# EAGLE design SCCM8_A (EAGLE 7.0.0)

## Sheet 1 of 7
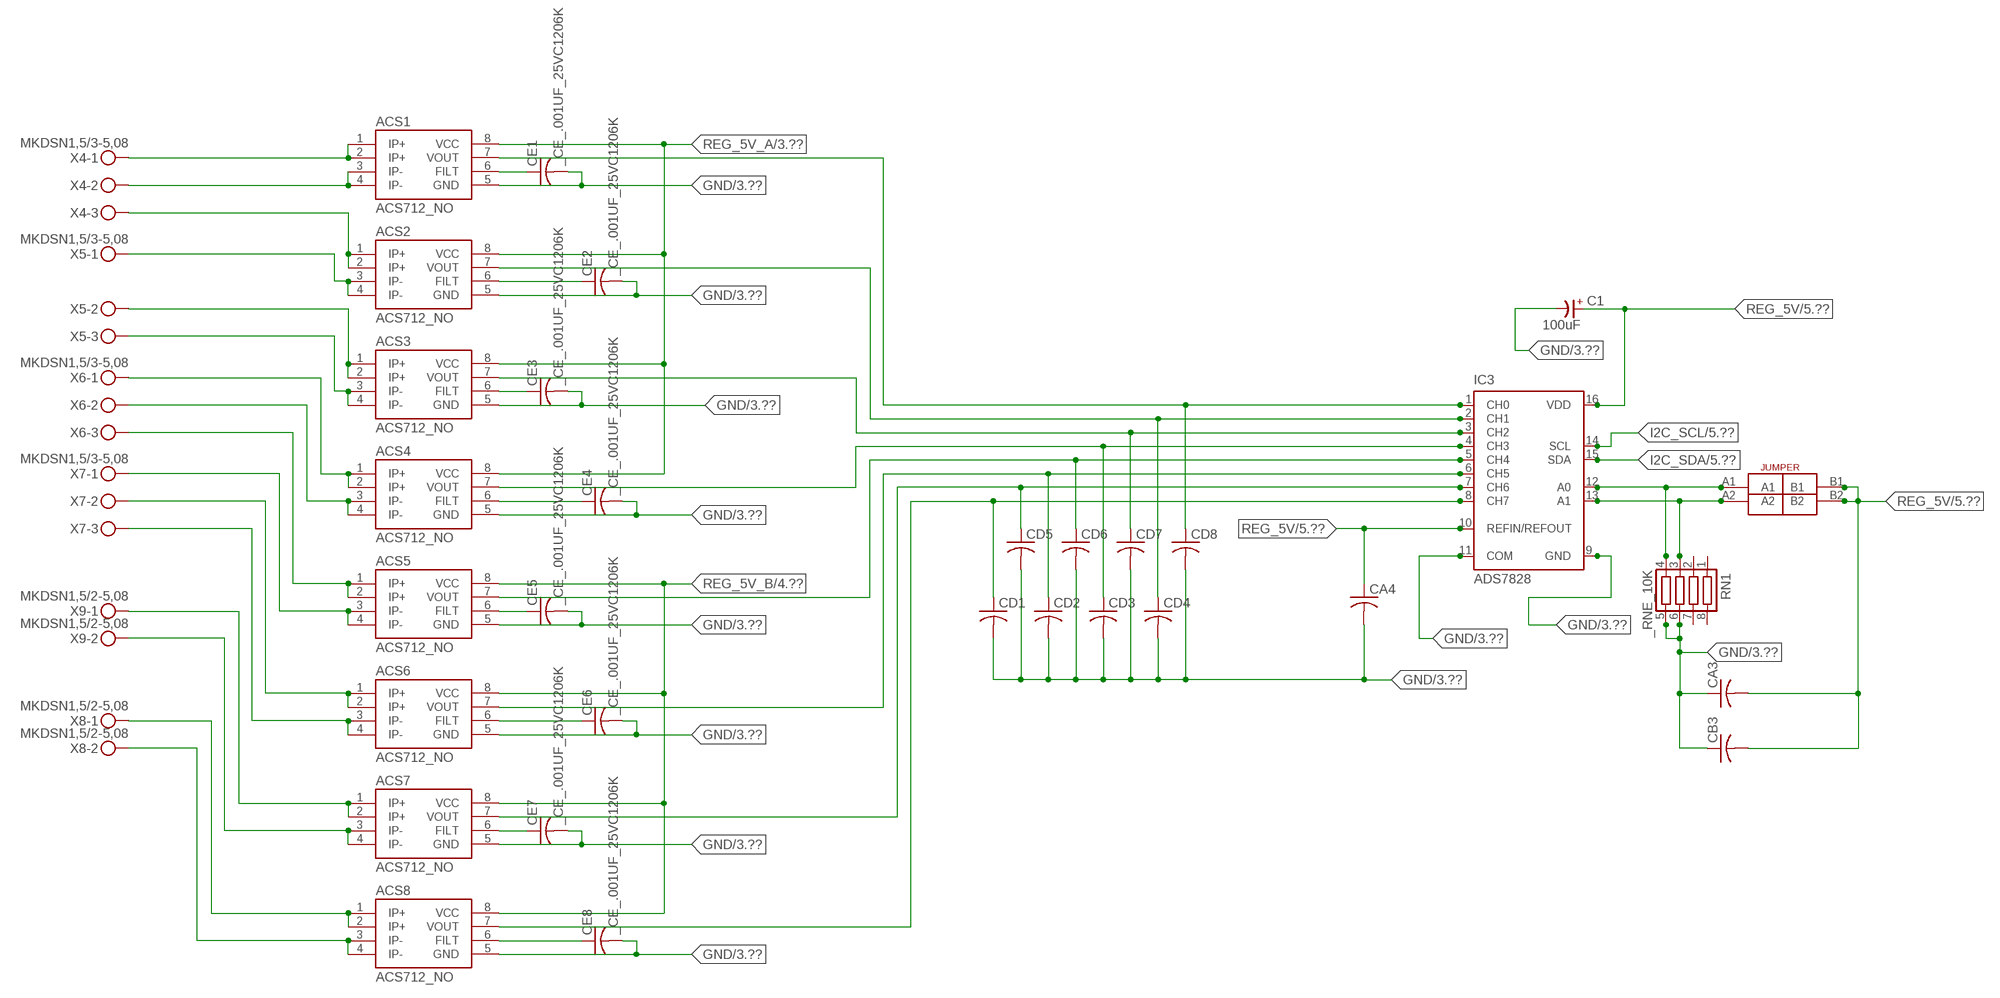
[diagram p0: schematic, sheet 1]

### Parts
ACS1  ACS712_NO  [_MA_DUAL_N-FET]
ACS2  ACS712_NO  [_MA_DUAL_N-FET]
ACS3  ACS712_NO  [_MA_DUAL_N-FET]
ACS4  ACS712_NO  [_MA_DUAL_N-FET]
ACS5  ACS712_NO  [_MA_DUAL_N-FET]
ACS6  ACS712_NO  [_MA_DUAL_N-FET]
ACS7  ACS712_NO  [_MA_DUAL_N-FET]
ACS8  ACS712_NO  [_MA_DUAL_N-FET]
C1  100uF  CP-E-025X060  [E-025X060]
CA3  CC1206KRX7R9BB104C1206K  [CC1206KRX7R9BB104]
CA4  CC1206KRX7R9BB104C1206K  [CC1206KRX7R9BB104]
CB3  TMK316F106ZL-TC1206K  [TMK316F106ZL-T]
CD1  _CD_10NF_50VC1206K  [_CD_10NF_50V]
CD2  _CD_10NF_50VC1206K  [_CD_10NF_50V]
CD3  _CD_10NF_50VC1206K  [_CD_10NF_50V]
CD4  _CD_10NF_50VC1206K  [_CD_10NF_50V]
CD5  _CD_10NF_50VC1206K  [_CD_10NF_50V]
CD6  _CD_10NF_50VC1206K  [_CD_10NF_50V]
CD7  _CD_10NF_50VC1206K  [_CD_10NF_50V]
CD8  _CD_10NF_50VC1206K  [_CD_10NF_50V]
CE1  _CE_.001UF_25VC1206K  [CE]
CE2  _CE_.001UF_25VC1206K  [CE]
CE3  _CE_.001UF_25VC1206K  [CE]
CE4  _CE_.001UF_25VC1206K  [CE]
CE5  _CE_.001UF_25VC1206K  [CE]
CE6  _CE_.001UF_25VC1206K  [CE]
CE7  _CE_.001UF_25VC1206K  [CE]
CE8  _CE_.001UF_25VC1206K  [CE]
IC3  ADS7828  [TSSOP16-PW]
RN1  _RNE_10K  [RNE]
U$4  JUMPER_2X2  [JUMPER_2X2]
X4  MKDSN1,5/3-5,08  [MKDSN1,5/3-5,08]
X5  MKDSN1,5/3-5,08  [MKDSN1,5/3-5,08]
X6  MKDSN1,5/3-5,08  [MKDSN1,5/3-5,08]
X7  MKDSN1,5/3-5,08  [MKDSN1,5/3-5,08]
X8  MKDSN1,5/2-5,08  [MKDSN1,5/2-5,08]
X9  MKDSN1,5/2-5,08  [MKDSN1,5/2-5,08]

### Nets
GND: ACS1.5(GND) ACS2.5(GND) ACS3.5(GND) ACS4.5(GND) ACS5.5(GND) ACS6.5(GND) ACS7.5(GND) ACS8.5(GND) C1.- CA3.1 CA4.2 CB3.1 CD1.2 CD2.2 CD3.2 CD4.2 CD5.2 CD6.2 CD7.2 CD8.2 CE1.2 CE2.2 CE3.2 CE4.2 CE5.2 CE6.2 CE7.2 CE8.2 IC3.9(GND) IC3.11(COM) RN1.5 RN1.6 ; also sheet 3,4,5,7
I2C_SCL: IC3.14(SCL) ; also sheet 5
I2C_SDA: IC3.15(SDA) ; also sheet 5
N$6: ACS5.7(VOUT) CD6.1 IC3.5(CH4)
N$7: ACS1.1(IP+) ACS1.2(IP+) X4.1
N$8: ACS1.3(IP-) ACS1.4(IP-) X4.2
N$9: ACS1.7(VOUT) CD8.1 IC3.1(CH0)
N$10: ACS2.7(VOUT) CD4.1 IC3.2(CH1)
N$11: ACS3.7(VOUT) CD7.1 IC3.3(CH2)
N$12: ACS4.7(VOUT) CD3.1 IC3.4(CH3)
N$13: ACS2.1(IP+) ACS2.2(IP+) X4.3
N$14: ACS6.7(VOUT) CD2.1 IC3.6(CH5)
N$15: ACS7.7(VOUT) CD5.1 IC3.7(CH6)
N$16: ACS2.3(IP-) ACS2.4(IP-) X5.1
N$17: IC3.12(A0) RN1.4 U$4.A1
N$18: IC3.13(A1) RN1.3 U$4.A2
N$19: ACS3.1(IP+) ACS3.2(IP+) X5.2
N$20: ACS3.3(IP-) ACS3.4(IP-) X5.3
N$21: ACS4.1(IP+) ACS4.2(IP+) X6.1
N$22: ACS4.3(IP-) ACS4.4(IP-) X6.2
N$23: ACS5.1(IP+) ACS5.2(IP+) X6.3
N$24: ACS5.3(IP-) ACS5.4(IP-) X7.1
N$25: ACS6.1(IP+) ACS6.2(IP+) X7.2
N$26: ACS6.3(IP-) ACS6.4(IP-) X7.3
N$27: ACS7.1(IP+) ACS7.2(IP+) X9.1
N$28: ACS7.3(IP-) ACS7.4(IP-) X9.2
N$29: ACS8.1(IP+) ACS8.2(IP+) X8.1
N$30: ACS8.3(IP-) ACS8.4(IP-) X8.2
N$33: ACS1.6(FILT) CE1.1
N$34: ACS2.6(FILT) CE2.1
N$35: ACS3.6(FILT) CE3.1
N$36: ACS4.6(FILT) CE4.1
N$37: ACS8.7(VOUT) CD1.1 IC3.8(CH7)
N$38: ACS5.6(FILT) CE5.1
N$39: ACS6.6(FILT) CE6.1
N$40: ACS7.6(FILT) CE7.1
N$41: ACS8.6(FILT) CE8.1
REG_5V: C1.+ CA3.2 CA4.1 CB3.2 IC3.10(REFIN/REFOUT) IC3.16(VDD) U$4.B1 U$4.B2 ; also sheet 5,7
REG_5V_A: ACS1.8(VCC) ACS2.8(VCC) ACS3.8(VCC) ACS4.8(VCC) ; also sheet 3
REG_5V_B: ACS5.8(VCC) ACS6.8(VCC) ACS7.8(VCC) ACS8.8(VCC) ; also sheet 4
Unconnected: RN1.1 RN1.2 RN1.7 RN1.8

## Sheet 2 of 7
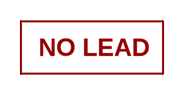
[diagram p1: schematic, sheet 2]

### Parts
U$16  NOPB_LOGO_SYM  [NOPB_LOGO_SYM]

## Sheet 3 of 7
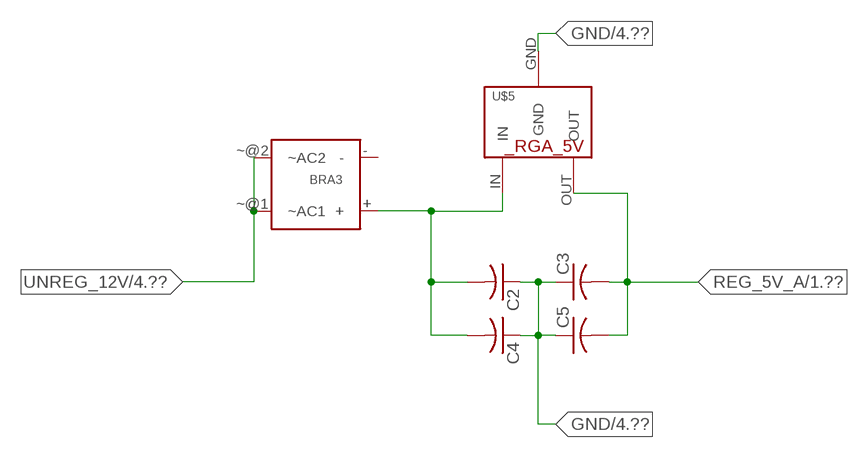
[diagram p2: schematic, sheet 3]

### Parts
BRA3  MB2S_  [MB2S]
C2  _CA_.10UF_50VC1206K  [_CA_.1UF_50V]
C3  _CA_.10UF_50VC1206K  [_CA_.1UF_50V]
C4  _CB_10UF_25VC1206K  [_CB_10UF_25V]
C5  _CB_10UF_25VC1206K  [_CB_10UF_25V]
U$5  _RGA_5V  [_RGA_5V]

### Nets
GND: C2.1 C3.1 C4.1 C5.1 U$5.GND ; also sheet 1,4,5,7
N$31: BRA3.+ C2.2 C4.2 U$5.IN
REG_5V_A: C3.2 C5.2 U$5.OUT ; also sheet 1
UNREG_12V: BRA3.~@1(~AC1) BRA3.~@2(~AC2) ; also sheet 4,5
Unconnected: BRA3.-

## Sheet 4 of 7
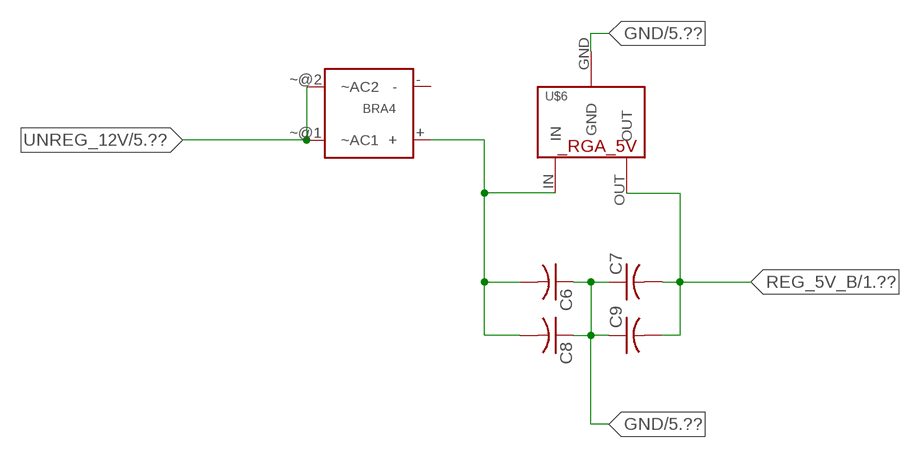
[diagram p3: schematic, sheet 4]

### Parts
BRA4  MB2S_  [MB2S]
C6  _CA_.10UF_50VC1206K  [_CA_.1UF_50V]
C7  _CA_.10UF_50VC1206K  [_CA_.1UF_50V]
C8  _CB_10UF_25VC1206K  [_CB_10UF_25V]
C9  _CB_10UF_25VC1206K  [_CB_10UF_25V]
U$6  _RGA_5V  [_RGA_5V]

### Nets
GND: C6.1 C7.1 C8.1 C9.1 U$6.GND ; also sheet 1,3,5,7
N$32: BRA4.+ C6.2 C8.2 U$6.IN
REG_5V_B: C7.2 C9.2 U$6.OUT ; also sheet 1
UNREG_12V: BRA4.~@1(~AC1) BRA4.~@2(~AC2) ; also sheet 3,5
Unconnected: BRA4.-

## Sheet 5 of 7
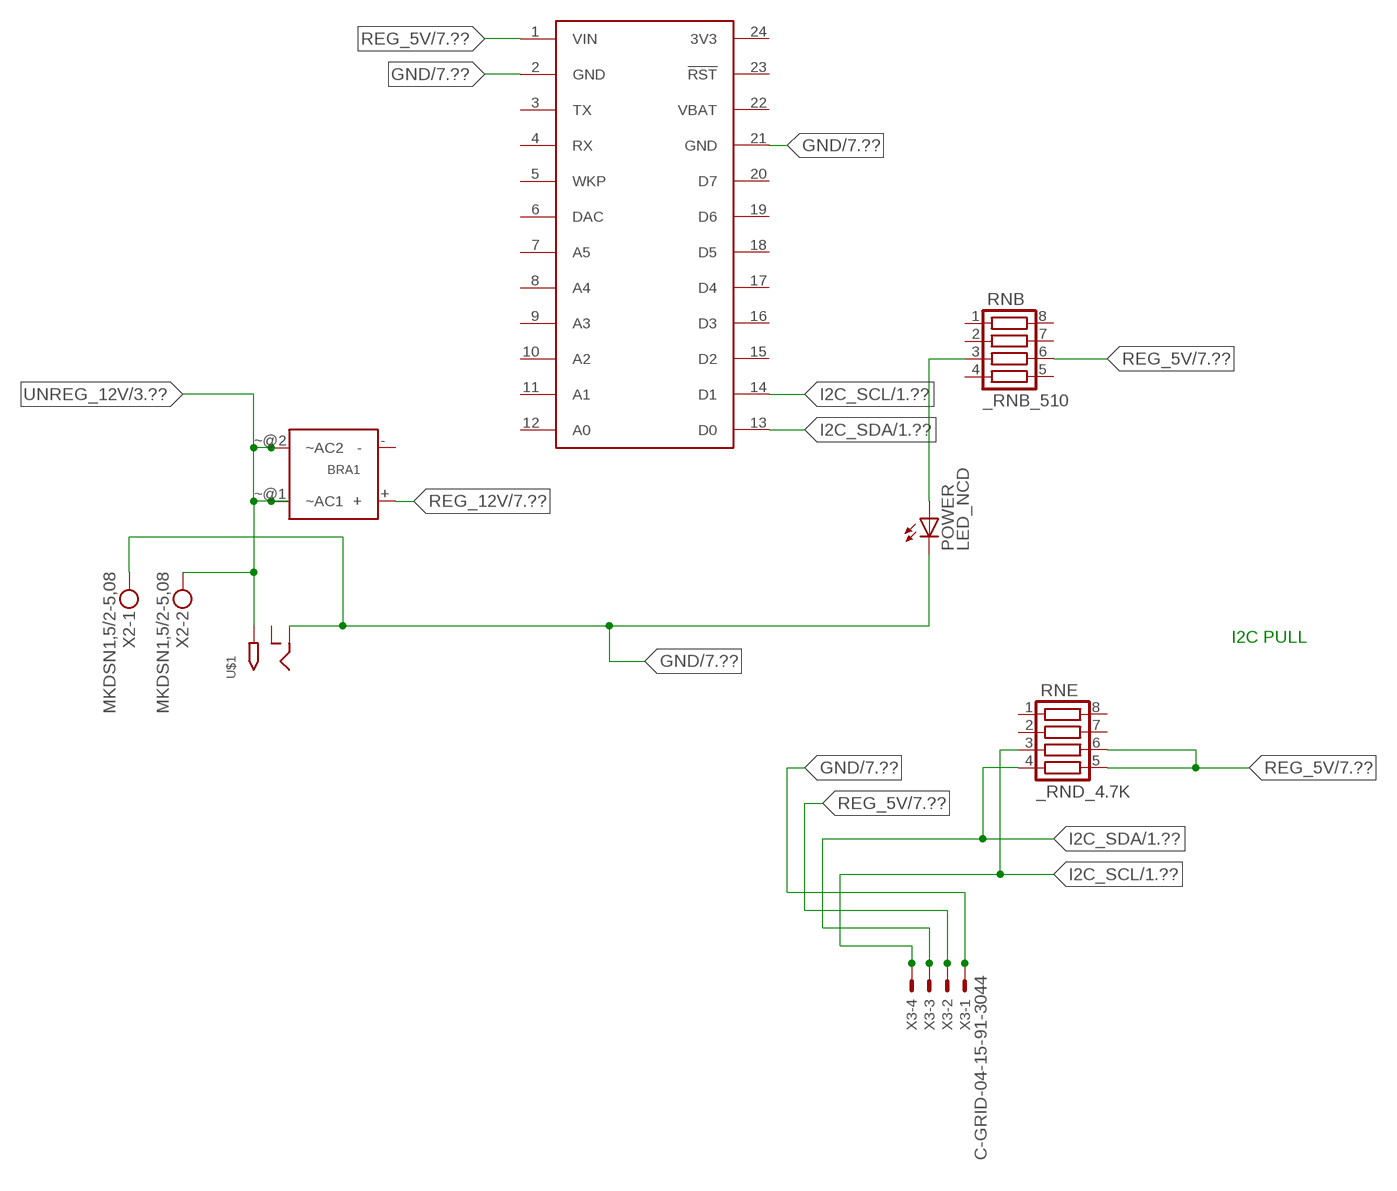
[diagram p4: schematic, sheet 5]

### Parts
BRA1  MB2S_  [MB2S]
POWER  LED_NCD  [CHIPLED_0603]
RNB  _RNB_510  [RNB]
RNE  _RND_4.7K  [RND]
S1  SPARK_CORECORE  [SPARK_CORE]
U$1  2.1MMJACK  [PJ-102A]
X2  MKDSN1,5/2-5,08  [MKDSN1,5/2-5,08]
X3  C-GRID-04-15-91-3044  [15-91-04]

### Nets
GND: POWER.C S1.2(GND) S1.21(GND) U$1.RING X2.1 X3.1 ; also sheet 1,3,4,7
I2C_SCL: RNE.3 S1.14(D1) X3.4 ; also sheet 1
I2C_SDA: RNE.4 S1.13(D0) X3.3 ; also sheet 1
N$2: POWER.A RNB.3
REG_5V: RNB.6 RNE.5 RNE.6 S1.1(VIN) X3.2 ; also sheet 1,7
REG_12V: BRA1.+ ; also sheet 7
UNREG_12V: BRA1.~@1(~AC1) BRA1.~@2(~AC2) U$1.TIP X2.2 ; also sheet 3,4
Unconnected: BRA1.- RNB.1 RNB.2 RNB.4 RNB.5 RNB.7 RNB.8 RNE.1 RNE.2 RNE.7 RNE.8 S1.3(TX) S1.4(RX) S1.5(WKP) S1.6(DAC) S1.7(A5) S1.8(A4) S1.9(A3) S1.10(A2) S1.11(A1) S1.12(A0) S1.15(D2) S1.16(D3) S1.17(D4) S1.18(D5) S1.19(D6) S1.20(D7) S1.23(!RST) U$1.RING_SW

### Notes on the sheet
- I2C PULL

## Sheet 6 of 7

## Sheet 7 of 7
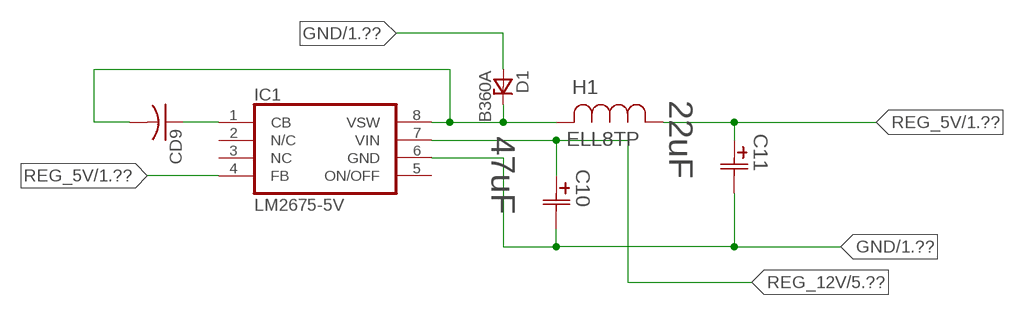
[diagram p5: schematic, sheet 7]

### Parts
C10  47uF  490-5463-6-NDCAP  [C2917(7343)-Y]
C11  22uF  490-5463-6-NDCAP  [C2917(7343)-Y]
CD9  _CD_10NF_50VC1206K  [_CD_10NF_50V]
D1  B360A  [DO214AC_ZENER]
H1  ELL8TP  [IND_ELL8TP]
IC1  LM2675-5V  LM2675  [SO-8]

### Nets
GND: C10.2(C2) C11.2(C2) D1.A IC1.6(GND) ; also sheet 1,3,4,5
N$1: CD9.2 D1.C H1.2 IC1.8(VSW)
N$3: CD9.1 IC1.1(CB)
REG_5V: C11.1(C1) H1.1 IC1.4(FB) ; also sheet 1,5
REG_12V: C10.1(C1) IC1.7(VIN) ; also sheet 5
Unconnected: IC1.2(N/C) IC1.5(ON/OFF)

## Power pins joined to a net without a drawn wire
3V3: S1.24(3V3)
NC: IC1.3(NC)
VBAT: S1.22(VBAT)

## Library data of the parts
ACS1-ACS8 = NCD_ULTIMATE_LIBRARY:ACS712_NO: Semiconductor Sensor Current Hall-effect-based isolated linear current sensor Digikey 620-1190-2-ND/ACS712ELCTR-20A-T
BRA1 BRA3 BRA4 = NCD_ULTIMATE_LIBRARY:MB2S: Bridge Rectifier BRA MB2S 200V 500ma Digikey MB2S-TPMSTR-ND/MB2S-TP
C1 = NCD_ULTIMATE_LIBRARY:CP-: Capacitors All Kinds POLARIZED CAP
C2 C3 C6 C7 = NCD_ULTIMATE_LIBRARY:_CA_.10UF_50V: Capacitor .1uF SMT
C4 C5 C8 C9 = NCD_ULTIMATE_LIBRARY:_CB_10UF_25V: Capacitor 10uF SMT
C10 C11 = NCD_ULTIMATE_bhaskar:490-5463-6-ND: NCD CAP
CA3 CA4 = NCD_ULTIMATE_LIBRARY:CC1206KRX7R9BB104: Capacitor CA .1uF 50V SMT C1206K CC1206KRX7R9BB104
CB3 = NCD_ULTIMATE_LIBRARY:TMK316F106ZL-T: Capacitor CB 10uF SMT 1206 TMK316F106ZL-T
CD1-CD9 = NCD_ULTIMATE_LIBRARY:_CD_10NF_50V: Capacitor 10nF SMT
CE1-CE8 = NCD_ULTIMATE_LIBRARY:_CE_.001UF_25V: Capacitor .001uF SMT
D1 = NCD_ULTIMATE_bhaskar:B360A: NCD DIODE B350A/B360A
H1 = NCD_ULTIMATE_bhaskar:ELL8TP: NCD coil
IC1 = NCD_ULTIMATE_bhaskar:LM2675: LM2675 NCD http://www.ti.com/lit/ds/symlink/lm2675.pdf
IC3 = NCD_ULTIMATE_LIBRARY:ADS7828: Semiconductor ADC I2C 12-Bit, 8-Channel Sampling ANALOG-TO-DIGITAL CONVERTER Digikey 296-12402-2-ND Source: www.ti.com .. ADS7828.pdf / ADS7828E/250; MF: TEXAS INSTRUMENTS; MPN: ADS7828E/250; OC_FARNELL: 1470338; OC_NEWARK: 74C7158
POWER = NCD_ULTIMATE_bhaskar:LED_NCD
RN1 = NCD_ULTIMATE_LIBRARY:_RNE_10K: Resistor Array RNE SMT 10K x 4 Single Resistor Source: http://www.ctscorp.com/components/Datasheets/CTSChipArrayDs.pdf Digikey 742C083103JPTR-ND/742C083103JP; OC_FARNELL: unknown; OC_NEWARK: unknown
RNB = NCD_ULTIMATE_LIBRARY:_RNB_510: Resistor Array RNB SMT 510 x 4 Single Resistor Source: http://www.ctscorp.com/components/Datasheets/CTSChipArrayDs.pdf Digikey 742C083511JPTR-ND/ 742C083511JP; OC_FARNELL: unknown; OC_NEWARK: unknown
RNE = NCD_ULTIMATE_LIBRARY:_RND_4.7K: Resistor Array RND SMT 4.7K x 4 Single Resistor Source: http://www.ctscorp.com/components/Datasheets/CTSChipArrayDs.pdf Digikey 742C083472JPTR-ND/742C083472JP; OC_FARNELL: unknown; OC_NEWARK: unknown
S1 = Spark:SPARK_CORE
U$1 = NCD_ULTIMATE_CONNECTORS:2.1MMJACK: 2.1mm x 5.5mm DC jack with internal switch. Digikey part #PJ-102A, 4UCON part #05537 By microbuilder.eu
U$4 = NCD_ULTIMATE_CONNECTORS:JUMPER_2X2
U$5 U$6 = NCD_ULTIMATE_LIBRARY:_RGA_5V: Regulator Linear 5V Digikey 497-7255-2-ND/ L7805CDT-TR
U$16 = PatternAgents-Logos:NOPB_LOGO_SYM: NOPB_LOGO_SYM
X2 X8 X9 = NCD_ULTIMATE_CONNECTORS:MKDSN1,5/2-5,08: MKDSN 1,5/ 2-5,08 Printklemme
X3 = NCD_ULTIMATE_CONNECTORS:C-GRID-04: CONNECTOR 4-Pos I2C wire to board 2.54 mm (0.100") pitch header Digikey WM1342-ND/0015912045; OC_FARNELL: unknown; OC_NEWARK: unknown
X4-X7 = NCD_ULTIMATE_CONNECTORS:MKDSN1,5/3-5,08: MKDSN 1,5/ 3-5,08 Printklemme Nennstrom: 13,5 A Nennspannung: 250 V Rastermaß: 5,08 mm Polzahl: 3 Anschlussart: Schraubanschluss Montage: Löten Anschlussrichtung Leiter/Platine: 0 ° Artikelnummer: 1729131 Source: http://eshop.phoenixcontact.com .. 1729131.pdf

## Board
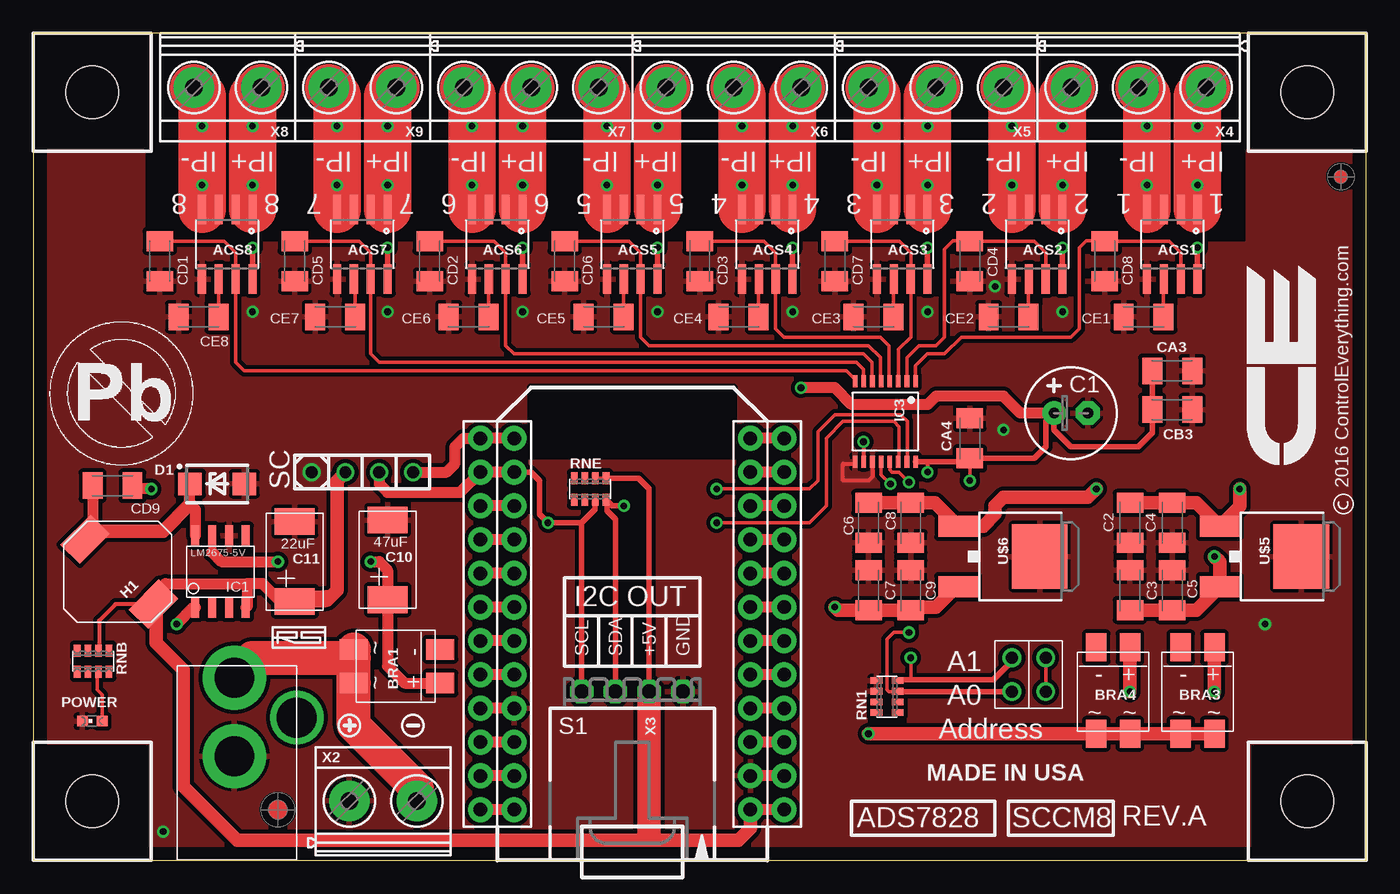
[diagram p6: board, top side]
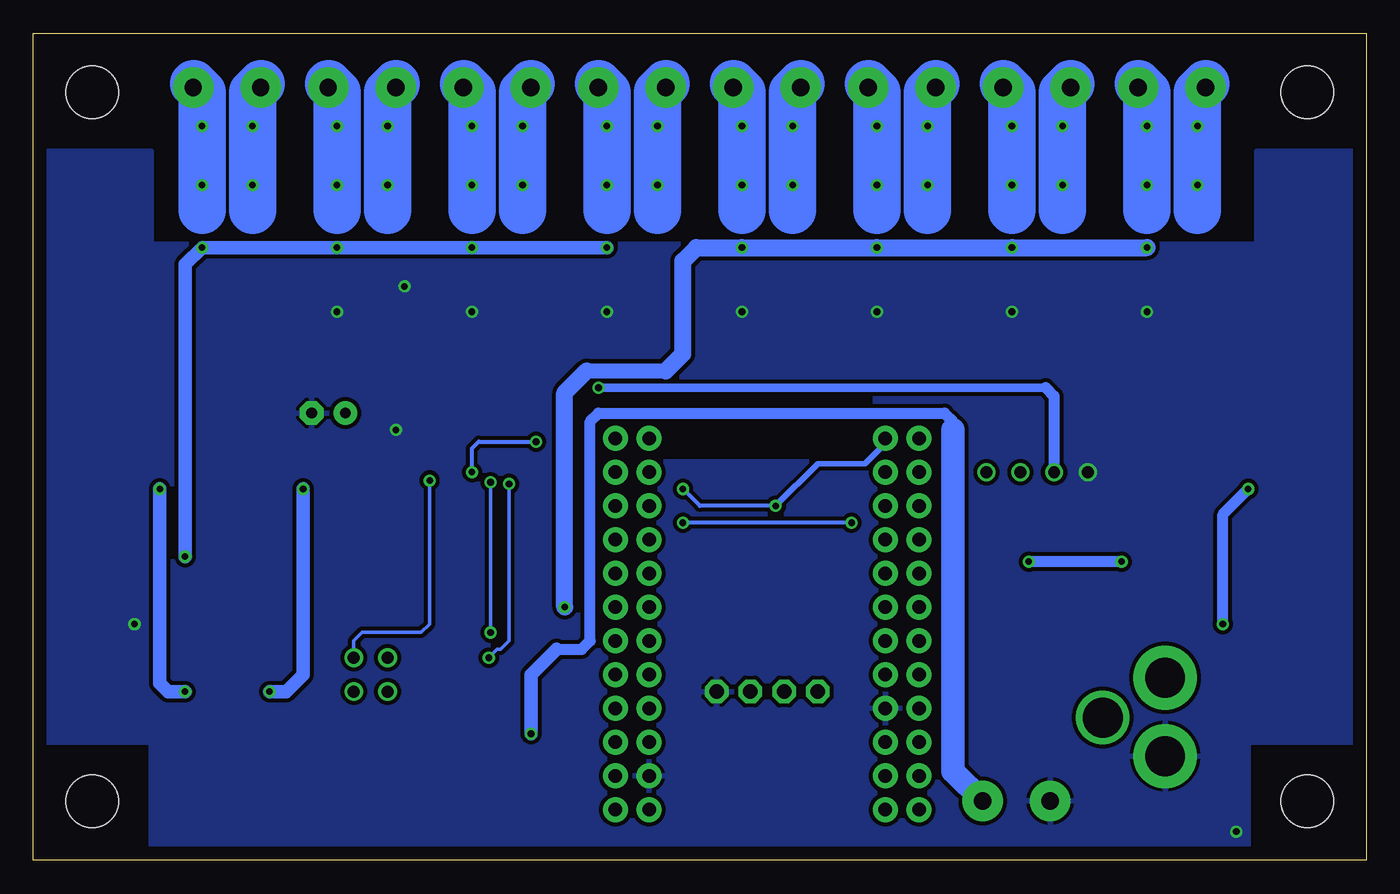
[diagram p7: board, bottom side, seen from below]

Size 100.33 x 62.23 mm. Coordinates in mm from the lower left corner, seen from the top.
Outline: 99.06,0 100.31,0
Outline: 0,61.9 0,60.96
Outline: 0,60.96 0,0 99.06,0
Outline: 99.06,0 100.33,0 100.33,62.23 0,62.23 0,60.96
Copper layers (1*16): Top 0.035mm / dielectric 1.5mm / Bottom 0.035mm
Design rules "default": minimum track width 10mil, minimum drill 24mil, track to track 8mil, track to pad 8mil, pad to pad 8mil, via to via 8mil, smd to smd 8mil, copper to edge 40mil, drill to drill 8mil, minimum pad ring 10mil, minimum via ring 8mil, stop-mask expansion 4mil, vias tented up to drill 0mil, thermal gap 10mil
Holes 3.96 mm at 4.45,4.45 95.89,4.45 95.89,57.78 4.45,57.78 4.45,4.45

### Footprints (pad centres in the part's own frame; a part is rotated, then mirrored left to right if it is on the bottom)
_MA_DUAL_N-FET = smd 0.61 x 2.21: 1 -1.905,-2.616; 2 -0.635,-2.616; 3 0.635,-2.616; 4 1.905,-2.616; 5 1.905,2.616; 6 0.635,2.616; 7 -0.635,2.616; 8 -1.905,2.616
MB2S = smd 1.55 x 2.1: + 0,-6.5; - 2.54,-6.5; ~@1 0,0; ~@2 2.54,0
E-025X060 = drill 0.813 pad 1.778: + -1.27,0 | drill 0.813 pad 1.778 octagon: - 1.27,0
_CA_.1UF_50V = smd 1.5 x 2: 1 -1.5,0; 2 1.5,0
_CB_10UF_25V = smd 1.5 x 2: 1 -1.5,0; 2 1.5,0
C2917(7343)-Y = smd 2 x 3: 1 -3,0; 2 3,0
CC1206KRX7R9BB104 = smd 1.5 x 2: 1 -1.5,0; 2 1.5,0
TMK316F106ZL-T = smd 1.5 x 2: 1 -1.5,0; 2 1.5,0
_CD_10NF_50V = smd 1.5 x 2: 1 -1.5,0; 2 1.5,0
CE = smd 1.5 x 2: 1 -1.5,0; 2 1.5,0
DO214AC_ZENER = smd 1.8 x 1.7: A 2.05,0; C -2.05,0
IND_ELL8TP = smd 2.054 x 3.2 rotated 45: 1 -2.442,-2.696; 2 2.442,2.442
SO-8 = smd 0.6 x 1.55: 1 -1.905,-2.69; 2 -0.635,-2.69; 3 0.635,-2.69; 4 1.905,-2.69; 5 1.905,2.71; 6 0.635,2.71; 7 -0.635,2.71; 8 -1.905,2.71
TSSOP16-PW = smd 0.35 x 0.9: 1 -2.275,-3.025; 2 -1.625,-3.025; 3 -0.975,-3.025; 4 -0.325,-3.025; 5 0.325,-3.025; 6 0.975,-3.025; 7 1.625,-3.025; 8 2.275,-3.025; 9 2.275,3.025; 10 1.625,3.025; 11 0.975,3.025; 12 0.325,3.025; 13 -0.325,3.025; 14 -0.975,3.025; 15 -1.625,3.025; 16 -2.275,3.025
CHIPLED_0603 = smd 0.8 x 0.8: A 0,-0.75; C 0,0.75
RNE = smd 0.5 x 0.9: 1 -1.2,-0.8; 2 -0.4,-0.8; 3 0.4,-0.8; 4 1.2,-0.8; 5 1.2,0.8; 6 0.4,0.8; 7 -0.4,0.8; 8 -1.2,0.8
RNB = smd 0.5 x 0.9: 1 -1.2,-0.8; 2 -0.4,-0.8; 3 0.4,-0.8; 4 1.2,-0.8; 5 1.2,0.8; 6 0.4,0.8; 7 -0.4,0.8; 8 -1.2,0.8
RND = smd 0.5 x 0.9: 1 -1.2,-0.8; 2 -0.4,-0.8; 3 0.4,-0.8; 4 1.2,-0.8; 5 1.2,0.8; 6 0.4,0.8; 7 -0.4,0.8; 8 -1.2,0.8
SPARK_CORE = drill 1.016 pad 1.88: 1 -8.89,13.97; 2 -8.89,11.43; 3 -8.89,8.89; 4 -8.89,6.35; 5 -8.89,3.81; 6 -8.89,1.27; 7 -8.89,-1.27; 8 -8.89,-3.81; 9 -8.89,-6.35; 10 -8.89,-8.89; 11 -8.89,-11.43; 12 -8.89,-13.97; 13 8.89,-13.97; 14 8.89,-11.43; 15 8.89,-8.89; 16 8.89,-6.35; 17 8.89,-3.81; 18 8.89,-1.27; 19 8.89,1.27; 20 8.89,3.81; 21 8.89,6.35; 22 8.89,8.89; 23 8.89,11.43; 24 8.89,13.97; 25 -11.43,13.97; 26 -11.43,11.43; 27 -11.43,8.89; 28 -11.43,6.35; 29 -11.43,3.81; 30 -11.43,1.27; 31 -11.43,-1.27; 32 -11.43,-3.81; 33 -11.43,-6.35; 34 -11.43,-8.89; 35 -11.43,-11.43; 36 -11.43,-13.97; 37 11.43,13.97; 38 11.43,11.43; 39 11.43,8.89; 40 11.43,6.35; 41 11.43,3.81; 42 11.43,1.27; 43 11.43,-1.27; 44 11.43,-3.81; 45 11.43,-6.35; 46 11.43,-8.89; 47 11.43,-11.43; 48 11.43,-13.97
PJ-102A = drill 3 pad 4.8: RING 0.1,-3.39; TIP 0.1,-9.29 | drill 3 pad 3.251: RING_SW -4.6,-6.29
JUMPER_2X2 = drill 0.9: A1 0,2.54; A2 0,0; B1 2.54,2.54; B2 2.54,0
_RGA_5V = smd 4.826 x 4.191: GND 0,2.096 | smd 1.6 x 3: IN -2.28,-4.04; OUT 2.28,-4.04
MKDSN1,5/2-5,08 = drill 1.3 pad 3.048: 1 -2.561,0.025; 2 2.519,0.025
15-91-04 = drill 1.1 pad 1.778 octagon: 1 -3.81,-7.62; 2 -1.27,-7.62; 3 1.27,-7.62; 4 3.81,-7.62
MKDSN1,5/3-5,08 = drill 1.3 pad 3.048: 1 -7.641,0.025; 2 -2.561,0.025; 3 2.519,0.025

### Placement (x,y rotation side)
ACS1  85.72,46.35 180 top
ACS2  75.56,46.35 180 top
ACS3  65.41,46.35 180 top
ACS4  55.24,46.35 180 top
ACS5  45.09,46.35 180 top
ACS6  34.92,46.35 180 top
ACS7  24.77,46.35 180 top
ACS8  14.61,46.35 180 top
BRA1  24.13,13.34 90 top
BRA3  88.9,9.53 180 top
BRA4  82.55,9.53 180 top
C1  78.11,33.66 0 top
C2  82.55,25.4 90 top
C3  82.55,20.32 270 top
C4  85.72,25.4 90 top
C5  85.72,20.32 270 top
C6  62.87,25.4 90 top
C7  62.87,20.32 270 top
C8  66.04,25.4 90 top
C9  66.04,20.32 270 top
C10  26.67,22.61 90 top
C11  19.68,22.48 90 top
CA3  85.72,36.83 180 top
CA4  70.48,31.75 90 top
CB3  85.72,33.91 180 top
CD1  9.53,45.09 270 top
CD2  29.84,45.09 270 top
CD3  50.16,45.09 270 top
CD4  70.48,45.09 270 top
CD5  19.68,45.09 270 top
CD6  40.01,45.09 270 top
CD7  60.33,45.09 270 top
CD8  80.64,45.09 270 top
CD9  5.97,28.19 180 top
CE1  83.57,40.89 180 top
CE2  73.41,40.89 180 top
CE3  63.25,40.89 180 top
CE4  53.09,40.89 180 top
CE5  42.93,40.89 180 top
CE6  32.77,40.89 180 top
CE7  22.73,40.89 180 top
CE8  12.45,40.89 180 top
D1  13.84,28.32 0 top
H1  6.35,21.72 90 top
IC1  14.1,21.72 0 top
IC3  64.14,33.02 180 top
POWER  4.45,10.48 90 top
RN1  64.26,12.32 90 top
RNB  4.51,14.99 0 top
RNE  41.91,27.94 0 top
S1  45.09,17.78 180 top
U$1  15.24,4.45 180 top
U$4  73.66,12.7 0 top
U$5  93.34,22.86 270 top
U$6  73.66,22.86 270 top
U$10  [VISION_REF15]  18.41,3.81 0 top
U$16  1.04,29.29 0 top
U$19  [VISION_REF10]  98.42,51.44 0 top
U$21  [ICON_USA]  79.12,7.24 180 top
U$22  [ICON_MINUS]  28.57,10.16 180 top
U$24  [ICON_PLUS]  23.81,10.16 90 top
X2  26.35,4.45 0 top
X3  45.09,5.08 180 top
X4  80.64,58.17 180 top
X5  65.41,58.17 180 top
X6  50.16,58.17 180 top
X7  34.92,58.17 180 top
X8  14.61,58.17 180 top
X9  24.77,58.17 180 top

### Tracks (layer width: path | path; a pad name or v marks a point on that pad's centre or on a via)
GND  (via drill 0.5, 0.9)
  Top 0.305: IC3.11 63.16,28.87 62.87,28.57 60.96,28.57 60.96,29.84 61.71,29.84 IC3.9
  Top 0.61: C4.1 85.72,24.13 | C8.1 66.04,24.13
  other vias: 72.39,43.18 73.03,32.38 77.47,41.27 67.31,41.27 57.15,41.27 46.99,41.27 36.83,41.27 26.67,41.27 16.51,41.27 92.71,17.78 9.78,2.16 20.95,29.21
  pour Bottom (isolate 0.305): -0.64,8.89 -0.64,53.34 8.26,53.34 8.26,46.35 91.44,46.35 91.44,53.34 100.97,53.34 100.97,8.89 91.44,8.89 91.44,-0.63 8.89,-0.63 8.89,8.89
  pour Top (isolate 0.305): -1.91,53.34 8.26,53.34 8.26,46.35 91.44,46.35 91.44,53.34 102.87,53.34 102.87,8.89 91.44,8.89 91.44,-1.91 8.89,-1.91 8.89,8.89 -1.91,8.89
I2C_SCL  (via drill 0.5, 0.9)
  Top 0.254: IC3.14 65.15,30.04 65.15,32.64 64.77,33.02 60.96,33.02 59.69,31.75 59.69,26.67 58.42,25.4 v51.44,25.4
  Top 0.406: X3.4 41.27,25.4 | 41.27,25.4 42.29,26.42 42.29,27.12 RNE.3 | S1.14 37.47,29.21 38.1,28.57 38.1,26.04 v38.73,25.4 41.27,25.4
  Top 0.813: v26.04,29.21 26.04,28.32 26.67,27.69 32.13,27.69 33.66,29.21
  Bottom 0.305: v38.73,25.4 v51.44,25.4
I2C_SDA  (via drill 0.5, 0.9)
  Top 0.254: IC3.15 65.79,30.02 65.79,33.02 65.28,33.53 60.96,33.53 60.33,33.53 59.05,32.26 59.05,28.57 58.42,27.94 v51.44,27.94
  Top 0.406: X3.3 43.81,25.65 43.18,26.29 43.18,27.07 RNE.4 43.58,26.67 v44.45,26.67
  Top 0.813: v28.57,29.21 31.11,29.21 31.75,29.84 31.75,31.11 32.38,31.75 33.66,31.75
  Bottom 0.305: v44.45,26.67 50.16,26.67 v51.44,27.94
  Bottom 0.406: S1.13 36.2,31.37 37.72,29.84 41.27,29.84 v44.45,26.67
N$1
  Top 0.813: H1.2 3.88,24.77 | D1.C 11.79,26.78 12.19,26.38 IC1.8 | CD9.2 4.47,24.79 4.45,24.77
  Top 1.016: 3.88,24.77 4.45,24.77 9.78,24.77 11.79,26.78
N$2
  Top 0.254: POWER.A 5.2,12.46 4.83,12.83 4.83,14.1 RNB.3
  Top 0.406: 4.95,14.14 RNB.3
N$3  (via drill 0.5)
  Top 0.813: IC1.1 12.04,19.03 v10.79,17.78 | v8.89,27.94 7.72,27.94 CD9.1
  Bottom 0.813: v10.79,17.78 10.79,26.04 v8.89,27.94
N$6
  Top 0.254: CD6.1 44.85,46.59 45.72,45.72 ACS5.7 45.72,39.37 46.35,38.73 62.87,38.73 63.75,37.85 63.75,36.1 IC3.5
N$7  (via drill 0.5)
  Top 0.254: ACS1.2 ACS1.1
  Top 3.556: ACS1.1 v87.63,50.8 v87.63,55.24 87.63,57.48 X4.1
  Bottom 3.556: 87.63,48.89 v87.63,50.8 v87.63,55.24 87.63,57.78 88.27,58.42
N$8  (via drill 0.5)
  Top 0.254: ACS1.4 ACS1.3
  Top 3.556: ACS1.4 v83.82,50.8 v83.82,55.24 83.82,57.53 X4.2
  Bottom 3.556: 83.82,48.89 v83.82,50.8 v83.82,55.24 83.82,57.78 83.19,58.42
N$9
  Top 0.254: ACS1.7 86.36,45.72 85.5,46.59 CD8.1 80.62,46.61 79.25,46.61 78.74,46.1 78.74,40.01 78.11,39.37 69.85,39.37 68.58,38.1 67.31,38.1 66.41,37.2 IC3.1
N$10
  Top 0.254: ACS2.7 76.2,45.72 75.33,46.59 CD4.1 70.46,46.61 69.22,46.61 68.58,45.97 68.58,39.37 67.94,38.73 66.67,38.73 65.76,37.82 IC3.2
N$11
  Top 0.254: CD7.1 65.17,46.59 66.04,45.72 ACS3.7 66.04,39.37 65.11,38.44 IC3.3
N$12
  Top 0.254: CD3.1 55.02,46.59 55.88,45.72 ACS4.7 55.88,40.01 56.52,39.37 63.75,39.37 64.39,38.73 64.39,36.12 IC3.4
N$13  (via drill 0.5)
  Top 0.254: ACS2.2 ACS2.1
  Top 3.556: ACS2.1 v77.47,50.8 v77.47,55.24 77.47,57.48 X4.3
  Bottom 3.556: 77.47,48.89 v77.47,50.8 v77.47,55.24 77.47,57.78 78.11,58.42
N$14
  Top 0.254: CD2.1 34.7,46.59 35.56,45.72 ACS6.7 35.56,38.73 36.2,38.1 62.48,38.1 63.12,37.47 63.12,36.09 IC3.6
N$15
  Top 0.254: CD5.1 24.54,46.59 25.4,45.72 ACS7.7 25.4,38.1 26.04,37.47 61.98,37.47 62.48,36.96 62.48,36.07 IC3.7
N$16  (via drill 0.5)
  Top 0.254: ACS2.4 ACS2.3
  Top 3.556: ACS2.4 v73.66,50.8 v73.66,55.24 73.66,57.53 X5.1
  Bottom 3.556: 73.66,48.89 v73.66,50.8 v73.66,55.24 73.66,57.78 73.03,58.42
N$17  (via drill 0.5)
  Top 0.254: IC3.12 63.81,29.01 v64.52,28.32 | v66.04,15.24 66.04,13.59
  Top 0.406: U$4.A1 73.66,14.99 72.26,13.59 66.04,13.59 65.13,13.59 RN1.4
  Bottom 0.254: v64.52,28.32 64.52,16.51 65.15,15.88 65.41,15.88 v66.04,15.24
N$18  (via drill 0.5)
  Top 0.254: v65.91,17.14 64.77,17.14 64.26,16.64 64.26,12.83 64.39,12.7 65.04,12.7 RN1.3 | IC3.13 64.46,29.39 64.64,29.21 65.15,29.21 v65.91,28.45
  Top 0.406: U$4.A2 65.08,12.7 RN1.3
  Bottom 0.254: v65.91,28.45 v65.91,17.14
N$19  (via drill 0.5)
  Top 0.254: ACS3.2 ACS3.1
  Top 3.556: ACS3.1 v67.31,50.8 v67.31,55.24 67.31,57.48 X5.2
  Bottom 3.556: 67.31,48.89 v67.31,50.8 v67.31,55.24 67.31,57.78 67.94,58.42
N$20  (via drill 0.5)
  Top 0.254: ACS3.4 ACS3.3
  Top 3.556: ACS3.4 v63.5,50.8 v63.5,55.24 63.5,57.53 X5.3
  Bottom 3.556: 63.5,48.89 v63.5,50.8 v63.5,55.24 63.5,57.78 62.87,58.42
N$21  (via drill 0.5)
  Top 0.254: ACS4.2 ACS4.1
  Top 3.556: ACS4.1 v57.15,50.8 v57.15,55.24 57.15,57.48 X6.1
  Bottom 3.556: 57.15,48.89 v57.15,50.8 v57.15,55.24 57.15,57.78 57.78,58.42
N$22  (via drill 0.5)
  Top 0.254: ACS4.4 ACS4.3
  Top 3.556: ACS4.4 v53.34,50.8 v53.34,55.24 53.34,57.53 X6.2
  Bottom 3.556: 53.34,48.89 v53.34,50.8 v53.34,55.24 53.34,57.78 52.7,58.42
N$23  (via drill 0.5)
  Top 0.254: ACS5.2 ACS5.1
  Top 3.556: ACS5.1 v46.99,50.8 v46.99,55.24 46.99,57.48 X6.3
  Bottom 3.556: 46.99,48.89 v46.99,50.8 v46.99,55.24 46.99,57.78 47.62,58.42
N$24  (via drill 0.5)
  Top 0.254: ACS5.4 ACS5.3
  Top 3.556: ACS5.4 v43.18,50.8 v43.18,55.24 43.18,57.53 X7.1
  Bottom 3.556: 43.18,48.89 v43.18,50.8 v43.18,55.24 43.18,57.78 42.55,58.42
N$25  (via drill 0.5)
  Top 0.254: ACS6.2 ACS6.1
  Top 3.556: ACS6.1 v36.83,50.8 v36.83,55.24 36.83,57.48 X7.2
  Bottom 3.556: 36.83,48.89 v36.83,50.8 v36.83,55.24 36.83,57.78 37.47,58.42
N$26  (via drill 0.5)
  Top 0.254: ACS6.4 ACS6.3
  Top 3.556: ACS6.4 v33.02,50.8 v33.02,55.24 33.02,57.53 X7.3
  Bottom 3.556: 33.02,48.89 v33.02,50.8 v33.02,55.24 33.02,57.78 32.38,58.42
N$27  (via drill 0.5)
  Top 0.254: ACS7.2 ACS7.1
  Top 3.556: ACS7.1 v26.67,50.8 v26.67,55.24 26.67,57.48 X9.1
  Bottom 3.556: 26.67,48.89 v26.67,50.8 v26.67,55.24 26.67,57.78 27.3,58.42
N$28  (via drill 0.5)
  Top 0.254: ACS7.4 ACS7.3
  Top 3.556: ACS7.4 v22.86,50.8 v22.86,55.24 22.86,57.53 X9.2
  Bottom 3.556: 22.86,48.89 v22.86,50.8 v22.86,55.24 22.86,57.78 22.23,58.42
N$29  (via drill 0.5)
  Top 0.254: ACS8.2 ACS8.1
  Top 3.556: ACS8.1 v16.51,50.8 v16.51,55.24 16.51,57.48 X8.1
  Bottom 3.556: 17.14,58.42 16.51,57.78 v16.51,55.24 v16.51,50.8 16.51,48.89
N$30  (via drill 0.5)
  Top 0.254: ACS8.4 ACS8.3
  Top 3.556: ACS8.4 v12.7,50.8 v12.7,55.24 12.7,57.53 X8.2
  Bottom 3.556: 12.06,58.42 12.7,57.78 v12.7,55.24 v12.7,50.8 12.7,48.89
N$31  (via drill 0.5)
  Top 1.016: C2.2 C4.2 87.55,26.9 U$5.IN 90.81,26.64 v90.81,27.94 | BRA3.+ v88.9,12.7
  Bottom 1.016: v88.9,12.7 90.17,12.7 90.81,13.34 v90.81,27.94
N$32  (via drill 0.5)
  Top 1.016: C6.2 C8.2 67.86,26.9 U$6.IN 71.5,25.14 72.39,26.04 72.39,26.67 73.03,27.3 79.38,27.3 v80.01,27.94 | v82.55,12.7 BRA4.+
  Bottom 1.016: v80.01,27.94 80.01,13.97 81.28,12.7 v82.55,12.7
N$33
  Top 0.254: CE1.1 85.07,43.71 ACS1.6
N$34
  Top 0.254: CE2.1 74.91,43.71 ACS2.6
N$35
  Top 0.254: CE3.1 64.75,43.71 ACS3.6
N$36
  Top 0.254: CE4.1 54.59,43.71 ACS4.6
N$37
  Top 0.254: CD1.1 14.38,46.59 15.24,45.72 ACS8.7 15.24,37.47 15.88,36.83 61.21,36.83 61.85,36.2 61.85,36.06 IC3.8
N$38
  Top 0.254: CE5.1 44.43,43.71 ACS5.6
N$39
  Top 0.254: CE6.1 34.27,43.71 ACS6.6
N$40
  Top 0.254: CE7.1 24.23,43.64 ACS7.6
N$41
  Top 0.254: CE8.1 13.95,43.71 ACS8.6
REG_5V  (via drill 0.5, 0.9)
  Top 0.254: U$4.B2 U$4.B1 | v70.48,28.57 CA4.1 | RNE.6 RNE.5
  Top 0.305: IC3.16 67.16,30 67.31,29.84 v67.31,29.21 | v62.48,31.5 62.48,30.02 IC3.10 | H1.1 6.19,19.27 4.95,18.03 4.95,15.83 RNB.6
  Top 0.406: IC3.16 70.23,30 CA4.1 75.33,30.25 76.2,31.11 76.2,33.02 C1.+ 76.83,32.38 78.11,31.11 83.19,31.11 84.22,32.16 CB3.2 CA3.2 | RNE.5 45.55,28.74 46.35,27.94 X3.2
  Top 0.813: C1.+ 74.3,33.66 73.03,34.93 67.94,34.93 67.31,34.29 61.59,34.29 60.33,35.56 v57.78,35.56 | 16.13,20.83 9.96,20.83 H1.1 | 16.13,20.83 17.27,20.83 18.41,19.68 20.75,19.68 C11.1 | IC1.4 16.13,19.15 16.13,20.83
  Top 1.016: 46.35,2.16 46.35,1.52 | 46.35,1.52 15.37,1.52 11.3,5.59 11.3,14.35 9.27,16.38 9.27,18.41 H1.1 | 22.05,19.68 22.23,19.68 22.86,20.32 22.86,28.57 v23.5,29.21 | S1.1 53.98,2.41 53.09,1.52 46.35,1.52
  Top 1.27: 20.75,19.68 22.05,19.68
  Top 1.778: X3.2 46.35,2.16
  Bottom 0.254: U$4.B1 76.2,16.51 75.56,17.14 71.12,17.14 70.48,17.78 v70.48,28.57
  Bottom 0.305: v67.31,29.21 67.31,30.99 66.8,31.5 v62.48,31.5
  Bottom 0.635: v57.78,35.56 24.13,35.56
  Bottom 0.813: 24.13,35.56 23.5,34.93 v23.5,29.21
REG_5V_A  (via drill 0.5)
  Top 0.406: ACS1.8 v87.63,46.1 | ACS2.8 v77.47,46.1 | ACS3.8 v67.31,46.1 | ACS4.8 v57.15,46.1
  Top 1.016: C3.2 C5.2 87.55,18.82 U$5.OUT 89.31,22.46 v88.9,22.86
  Bottom 1.016: v88.9,22.86 88.9,44.83 v87.63,46.1 v77.47,46.1 v67.31,46.1 v57.15,46.1
REG_5V_B  (via drill 0.5)
  Top 0.406: ACS5.8 v46.99,46.1 | ACS6.8 v36.83,46.1 | ACS7.8 v26.67,46.1 | ACS8.8 v16.51,46.1
  Top 1.016: U$6.OUT 69.47,20.58 67.94,19.05 66.27,19.05 C9.2 C7.2 60.55,18.82 v60.33,19.05
  Bottom 1.143: 58.67,36.83 52.7,36.83
  Bottom 1.27: v60.33,19.05 60.33,35.18 58.67,36.83 | 52.7,36.83 51.44,38.1 51.44,45.09 50.42,46.1 v46.99,46.1 v36.83,46.1 v26.67,46.1 v16.51,46.1
REG_12V  (via drill 0.5)
  Top 0.61: IC1.7 13.46,23.16 | 14.1,22.48 14.15,22.48
  Top 0.813: v18.41,22.48 14.15,22.48 13.46,23.16 | v25.4,22.48 26.04,22.48 26.67,21.84 C10.1 26.67,14.61 27.94,13.34 BRA1.+
  Bottom 0.813: v18.41,22.48 v25.4,22.48
UNREG_12V  (via drill 0.5)
  Top 1.016: BRA4.~@2 BRA4.~@1 BRA3.~@2 BRA3.~@1 v62.87,9.53
  Top 2.54: X2.2 28.87,5.42 24.13,10.16 BRA1.~@1 24.13,15.24 | 24.13,15.24 BRA1.~@2 | U$1.TIP 15.14,13.87 16.51,15.24 24.13,15.24
  Bottom 0.813: 60.96,15.88 59.05,15.88 58.42,16.51 58.42,33.02 57.78,33.66 31.75,33.66 31.11,33.02 31.11,32.38
  Bottom 1.016: v62.87,9.53 62.87,13.97 60.96,15.88
  Bottom 1.778: 31.11,32.38 31.11,6.71 X2.2

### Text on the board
tNames: IP- | IP+ | IP- | IP+ | IP- | IP+ | IP- | IP+ | IP- | IP+ | IP- | IP+ | IP- | IP+ | IP- | IP+ | 8 | 8 | 7 | 7 | 6 | 6 | 5 | 5 | 4 | 4 | 3 | 3 | 2 | 2 | 1 | 1 | SC | 2016 ControlEverything.com | I2C OUT | SCL | SDA | +5V | GND | A1 | A0 | Address | REV.A | ADS7828 | SCCM8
